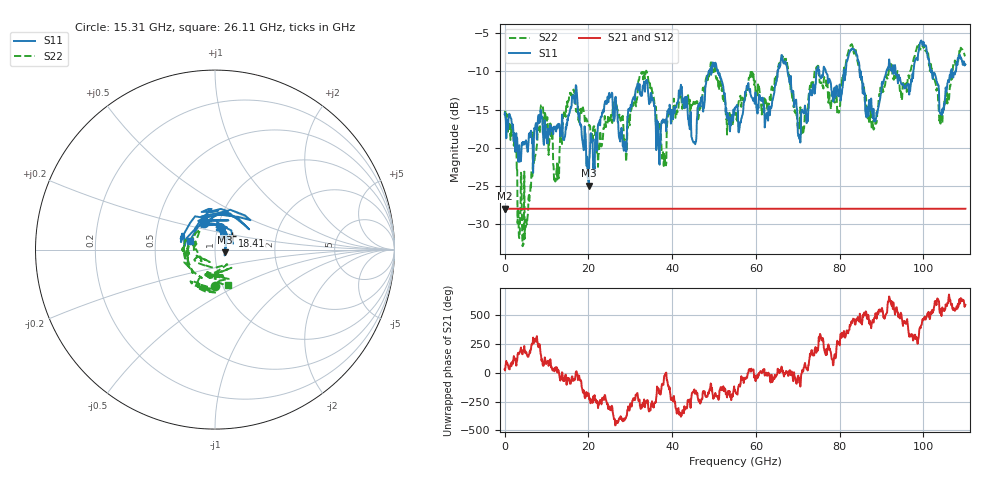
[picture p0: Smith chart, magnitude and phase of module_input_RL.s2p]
! Created with skrf 1.10.0 (http://scikit-rf.org).
# GHz S RI R 50.0
!freq ReS11 ImS11 ReS21 ImS21 ReS12 ImS12 ReS22 ImS22
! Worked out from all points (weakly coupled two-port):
!   1101 points, 10 MHz to 110 GHz, reference 50 ohm
!   highest |S21| = -27.96 dB at 110 MHz (marker M1); lowest = -28.0 dB at 10 MHz (marker M2)
!   lowest |S11| = -25.0 dB at 20.11 GHz (marker M3), VSWR 1.12, Z = 55.7 - j1.7 ohm
!   |S11| at or under -10 dB: start of sweep to 48.74 GHz; 50.94 GHz to 65.19 GHz (14.24 GHz wide, 24.5 % of centre); 67.56 GHz to 74.4 GHz (6.843 GHz wide, 9.64 % of centre)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
!   |S22| runs from -32.8 to -6.4 dB; largest |S21 - S12| = 0
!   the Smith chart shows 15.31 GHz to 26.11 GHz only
!   S11 on the Smith chart (normalised r, x): 15.31 GHz: 0.85, +0.26; 18.41 GHz: 1.20, +0.18; 26.11 GHz: 0.75, +0.07
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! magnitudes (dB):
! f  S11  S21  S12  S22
! 10 MHz  -15.6  -28.0  -28.0  -15.4
! 110 MHz  -15.4  -28.0  -28.0  -15.3
! 4.71 GHz  -19.6  -28.0  -28.0  -23.1
! 8.709 GHz  -15.3  -28.0  -28.0  -14.4
! 12.41 GHz  -17.1  -28.0  -28.0  -22.9
! 15.31 GHz  -15.8  -28.0  -28.0  -13.8
! 18.41 GHz  -18.3  -28.0  -28.0  -15.2
! 20.11 GHz  -25.0  -28.0  -28.0  -17.1
! 26.11 GHz  -16.5  -28.0  -28.0  -13.6
! 33.71 GHz  -11.3  -28.0  -28.0  -10.1
! 36.71 GHz  -17.0  -28.0  -28.0  -17.1
! 41.91 GHz  -12.8  -28.0  -28.0  -12.8
! 45.31 GHz  -19.3  -28.0  -28.0  -14.0
! 50.11 GHz  -9.4  -28.0  -28.0  -9.8
! 55.01 GHz  -14.9  -28.0  -28.0  -15.6
! 73.4 GHz  -13.1  -28.0  -28.0  -12.1
! 82.8 GHz  -7.1  -28.0  -28.0  -6.5
! 88.1 GHz  -14.9  -28.0  -28.0  -17.6
! 91.7 GHz  -9.3  -28.0  -28.0  -10.0
! 100.2 GHz  -6.6  -28.0  -28.0  -7.0
! 104.2 GHz  -15.6  -28.0  -28.0  -16.0
! 110 GHz  -9.1  -28.0  -28.0  -8.0
